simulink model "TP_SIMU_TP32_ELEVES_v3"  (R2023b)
settings: Solver=ode15s  StartTime=0.0  StopTime=6  RelTol=1e-3  EnableMultiTasking=on
libraries: fl_lib x24, nesl_utility x12, sdl_lib x2

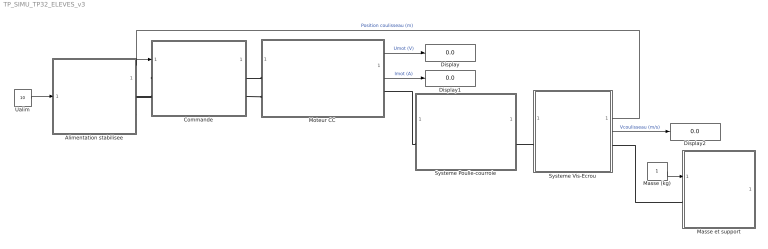
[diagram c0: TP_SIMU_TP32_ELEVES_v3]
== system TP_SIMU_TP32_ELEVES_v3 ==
  Alimentation stabilisee : Subsystem
  Commande : Subsystem
  Display : Display
  Display1 : Display
  Display2 : Display
  Masse (kg) : Constant
  Masse et support : Subsystem
  Moteur CC : Subsystem
  Systeme Poulie-courroie : Subsystem  mask{rend=0.64}
      mask prompts: rend "Rendement"
  Systeme Vis-Ecrou : Subsystem
  Ualim : Constant  Value=10
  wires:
  Masse (kg)/1 -> Masse et support/1(In1)
  Systeme Vis-Ecrou/1(Position coulisseau) -> Commande/1(In1)  "Position coulisseau (m)"
  Ualim/1 -> Alimentation stabilisee/1(Ualim)
  Moteur CC/1(Umot) -> Display/1  "Umot (V)"
  Moteur CC/2(Imot) -> Display1/1  "Imot (A)"
  Systeme Vis-Ecrou/2(Vcoulisseau) -> Display2/1  "Vcoulisseau (m/s)"
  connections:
  Systeme Poulie-courroie/LConn1 -- Moteur CC/RConn1
  Commande/RConn1 -- Moteur CC/LConn1
  Commande/LConn1 -- Alimentation stabilisee/RConn1
  Alimentation stabilisee/RConn2 -- Commande/LConn2
  Commande/RConn2 -- Moteur CC/LConn2
  Systeme Vis-Ecrou/LConn1 -- Systeme Poulie-courroie/RConn1
  Masse et support/LConn1 -- Systeme Vis-Ecrou/RConn1

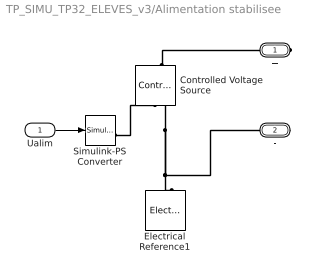
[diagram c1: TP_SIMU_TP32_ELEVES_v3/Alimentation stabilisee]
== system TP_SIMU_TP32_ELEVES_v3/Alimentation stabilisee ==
  Ualim : Inport
  Controlled Voltage Source : fl_lib/Electrical/Electrical Sources/Controlled Voltage Source
  Electrical Reference1 : fl_lib/Electrical/Electrical Elements/Electrical Reference
  Simulink-PS Converter : nesl_utility/Simulink-PS Converter  PhysicalDomain=network_engine_domain  SubClassName=ps_input  LeftPortType=input  RightPortType=output  PseudoPeriodic=off  Frequencies=[]  NoiseDistribution=none  NoiseParameters=[]  Unit=1  AffineConversion=off  FilteringAndDerivatives=provide  SimscapeFilterOrder=1  InputFilterTimeConstant=0.001  UdotUserProvided=0
  + : PMIOPort  Side=Right
  - : PMIOPort  Port=2  Side=Right
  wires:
  Ualim/1 -> Simulink-PS Converter/1
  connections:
  Controlled Voltage Source/LConn1 -- +/RConn1
  Electrical Reference1/LConn1 -- Controlled Voltage Source/RConn2 -- -/RConn1
  Simulink-PS Converter/RConn1 -- Controlled Voltage Source/RConn1

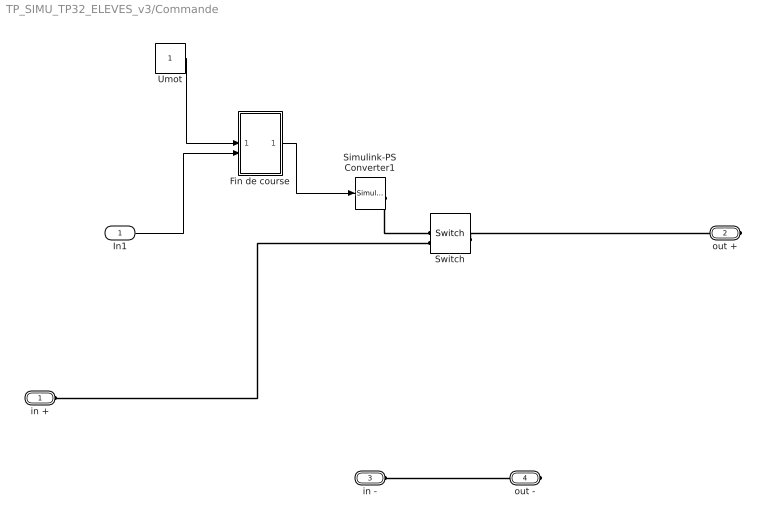
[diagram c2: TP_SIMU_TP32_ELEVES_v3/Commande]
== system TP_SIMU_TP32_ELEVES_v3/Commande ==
  In1 : Inport
  Fin de course : Subsystem
  Simulink-PS Converter1 : nesl_utility/Simulink-PS Converter  PhysicalDomain=network_engine_domain  SubClassName=ps_input  LeftPortType=input  RightPortType=output  PseudoPeriodic=off  Frequencies=[]  NoiseDistribution=none  NoiseParameters=[]  Unit=V  AffineConversion=off  FilteringAndDerivatives=zero  SimscapeFilterOrder=1  InputFilterTimeConstant=.001  UdotUserProvided=0
  Switch : fl_lib/Electrical/Electrical Elements/Switch  R_closed=0.01 Ohm  G_open=1e-8 1/Ohm  Threshold=0  i_specify=off  i_priority=None  i=0 A  i_nominal_specify=off  i_nominal_unit=A  i_nominal_value=1  v_specify=off  v_priority=None  v=0 V  v_nominal_specify=off  v_nominal_unit=V  v_nominal_value=1
  Umot : Constant
  in + : PMIOPort  Side=Left
  out + : PMIOPort  Port=2  Side=Right
  in - : PMIOPort  Port=3  Side=Left
  out - : PMIOPort  Port=4  Side=Right
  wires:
  Umot/1 -> Fin de course/1(In1)
  In1/1 -> Fin de course/2(In2)
  Fin de course/1(Out1) -> Simulink-PS Converter1/1
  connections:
  Switch/RConn2 -- in +/RConn1
  Simulink-PS Converter1/RConn1 -- Switch/RConn1
  Switch/LConn1 -- out +/RConn1
  in -/RConn1 -- out -/RConn1

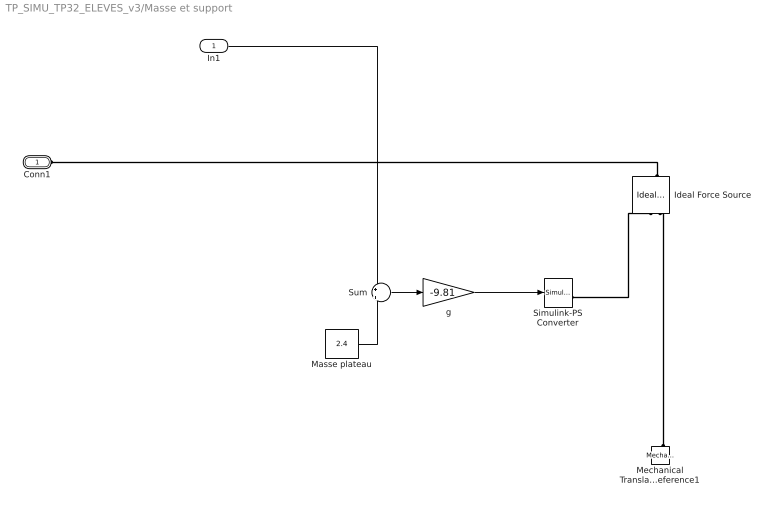
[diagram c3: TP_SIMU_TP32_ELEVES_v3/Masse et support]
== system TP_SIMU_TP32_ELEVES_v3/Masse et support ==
  In1 : Inport
  Ideal Force Source : fl_lib/Mechanical/Mechanical Sources/Ideal Force Source
  Masse plateau : Constant  Value=2.4
  Mechanical Translational Reference1 : fl_lib/Mechanical/Translational Elements/Mechanical Translational Reference
  Simulink-PS Converter : nesl_utility/Simulink-PS Converter  PhysicalDomain=network_engine_domain  SubClassName=ps_input  LeftPortType=input  RightPortType=output  PseudoPeriodic=off  Frequencies=[]  NoiseDistribution=none  NoiseParameters=[]  Unit=1  AffineConversion=off  FilteringAndDerivatives=zero  SimscapeFilterOrder=1  InputFilterTimeConstant=.001  UdotUserProvided=0
  Sum : Sum  Inputs=+|+
  g : Gain  Gain=-9.81
  Conn1 : PMIOPort  Side=Left
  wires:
  g/1 -> Simulink-PS Converter/1
  Sum/1 -> g/1
  Masse plateau/1 -> Sum/2
  In1/1 -> Sum/1
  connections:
  Mechanical Translational Reference1/LConn1 -- Ideal Force Source/RConn2
  Ideal Force Source/LConn1 -- Conn1/RConn1
  Simulink-PS Converter/RConn1 -- Ideal Force Source/RConn1

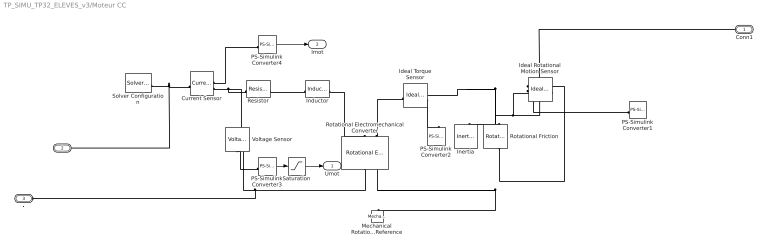
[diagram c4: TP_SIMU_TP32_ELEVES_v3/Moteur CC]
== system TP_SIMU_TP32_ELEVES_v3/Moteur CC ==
  Current Sensor : fl_lib/Electrical/Electrical Sensors/Current Sensor
  Ideal Rotational Motion Sensor : fl_lib/Mechanical/Mechanical Sensors/Ideal Rotational Motion Sensor  reference=foundation.enum.MeasurementReference.difference  acceleration_port=false  velocity_port=true  position_port=true  wrap_angle=false  offset=0 rad
  Ideal Torque Sensor : fl_lib/Mechanical/Mechanical Sensors/Ideal Torque Sensor
  Inductor : fl_lib/Electrical/Electrical Elements/Inductor  l=2e-4 H  r=0 Ohm  g=1e-9 1/Ohm  i_specify=off  i_priority=None  i=0 A  i_nominal_specify=off  i_nominal_unit=A  i_nominal_value=1  v_specify=off  v_priority=None  v=0 V  v_nominal_specify=off  v_nominal_unit=V  v_nominal_value=1  i_L_specify=on  i_L_priority=High  i_L=0 A  i_L_nominal_specify=off  i_L_nominal_unit=A  i_L_nominal_value=1
  Inertia : fl_lib/Mechanical/Rotational Elements/Inertia  inertia=5e-5 kg*m^2  num_ports=foundation.enum.numPorts2.one  w_specify=on  w_priority=High  w=0 rad/s  w_nominal_specify=off  w_nominal_unit=rad/s  w_nominal_value=1  t_specify=off  t_priority=None  t=0 N*m  t_nominal_specify=off  t_nominal_unit=N*m  t_nominal_value=1
  Mechanical Rotational Reference : fl_lib/Mechanical/Rotational Elements/Mechanical Rotational Reference
  PS-Simulink Converter1 : nesl_utility/PS-Simulink Converter  PhysicalDomain=network_engine_domain  SubClassName=ps_output  LeftPortType=input  RightPortType=output  PseudoPeriodic=off  Frequencies=[]  VectorFormat=1-D array  Unit=rad/s  AffineConversion=off
  PS-Simulink Converter2 : nesl_utility/PS-Simulink Converter  PhysicalDomain=network_engine_domain  SubClassName=ps_output  LeftPortType=input  RightPortType=output  PseudoPeriodic=off  Frequencies=[]  VectorFormat=1-D array  Unit=N*m  AffineConversion=off
  PS-Simulink Converter3 : nesl_utility/PS-Simulink Converter  PhysicalDomain=network_engine_domain  SubClassName=ps_output  LeftPortType=input  RightPortType=output  PseudoPeriodic=off  Frequencies=[]  VectorFormat=1-D array  Unit=V  AffineConversion=off
  PS-Simulink Converter4 : nesl_utility/PS-Simulink Converter  PhysicalDomain=network_engine_domain  SubClassName=ps_output  LeftPortType=input  RightPortType=output  PseudoPeriodic=off  Frequencies=[]  VectorFormat=1-D array  Unit=A  AffineConversion=off
  Resistor : fl_lib/Electrical/Electrical Elements/Resistor  R=1.8 Ohm  i_specify=off  i_priority=None  i=0 A  i_nominal_specify=off  i_nominal_unit=A  i_nominal_value=1  v_specify=off  v_priority=None  v=0 V  v_nominal_specify=off  v_nominal_unit=V  v_nominal_value=1
  Rotational Electromechanical Converter : fl_lib/Electrical/Electrical Elements/Rotational Electromechanical Converter  K=0.019 V/(rad/s)  i_specify=off  i_priority=None  i=0 A  i_nominal_specify=off  i_nominal_unit=A  i_nominal_value=1  v_specify=off  v_priority=None  v=0 V  v_nominal_specify=off  v_nominal_unit=V  v_nominal_value=1  t_specify=off  t_priority=None  t=0 N*m  t_nominal_specify=off  t_nominal_unit=N*m  t_nominal_value=1  w_specify=off  w_priority=None  w=0 rad/s  w_nominal_specify=off  w_nominal_unit=rad/s  w_nominal_value=1
  Rotational Friction : fl_lib/Mechanical/Rotational Elements/Rotational Friction  brkwy_trq=1.2e-2 N*m  brkwy_vel=0.060623 rad/s  Col_trq=1.2e-2 N*m  visc_coef=5e-9 N*m/(rad/s)  w_specify=off  w_priority=None  w=0 rad/s  w_nominal_specify=off  w_nominal_unit=rad/s  w_nominal_value=1  t_specify=off  t_priority=None  t=0 N*m  t_nominal_specify=off  t_nominal_unit=N*m  t_nominal_value=1
  Saturation : Saturate  UpperLimit=20
  Solver Configuration : nesl_utility/Solver Configuration  PhysicalDomain=network_engine_domain  SubClassName=solver  LeftPortType=input  RightPortType=generic  Tones=[]  Harmonics=[]  SimulateNoise=off  Profile=off  UseLocalSampling=off  EnableSwitchedLinearOptims=on  FrequencyDomain=off  UseCCode=off  RelTol=0.001  AbsTol=1e-06  MinStep=1e-09  ToWorkspace=off  RevertToSquareIcSolve=off  NumHomotopyIterations=100  PhasorMode=off  PhasorModeNumHarmonics=1  ConsistencySolver=NEWTON_FTOL  IndexReductionMethod=DerivativeReplacement  DoDC=off  ResidualTolerance=1e-9  ConsistencyTolSource=GLOBAL  ConsistencyAbsTol=0.001  ConsistencyRelTol=0.001  ConsistencyTolFactor=0.001  UseLocalSolver=off  LocalSolverChoice=NE_BACKWARD_EULER_ADVANCER  ResolveIndetEquations=on  FunctionEvalNumThread=1  LocalSolverSampleTime=.001  DoFixedCost=off  MaxNonlinIter=3  MaxModeIter=2  ComputeImpulses=off  ImpulseIterations=2  LinearAlgebra=Sparse  LinearAlgebraNumThread=0  EquationFormulation=NE_TIME_EF  DelaysMemoryBudget=1024  AutomaticFiltering=on  FilteringTimeConstant=0.001  PartitionStorageMethod=AS_NEEDED  PartitionMemoryBudget=1024  PartitionMethod=FAST  MultibodyUseLocalSolver=off  MultibodyLocalSolverChoice=ODE1  MultibodyLocalSolverSampleTime=0.001
  Voltage Sensor : fl_lib/Electrical/Electrical Sensors/Voltage Sensor
  Conn1 : PMIOPort  Side=Right
  + : PMIOPort  Port=2  Side=Left
  - : PMIOPort  Port=3  Side=Left
  Umot : Outport  VectorParamsAs1DForOutWhenUnconnected=off
  Imot : Outport  Port=2  VectorParamsAs1DForOutWhenUnconnected=off
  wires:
  PS-Simulink Converter3/1 -> Saturation/1
  PS-Simulink Converter4/1 -> Imot/1
  Saturation/1 -> Umot/1
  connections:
  Ideal Rotational Motion Sensor/RConn2 -- PS-Simulink Converter1/LConn1
  Current Sensor/RConn1 -- PS-Simulink Converter4/LConn1
  Rotational Friction/RConn1 -- Rotational Electromechanical Converter/RConn2 -- Mechanical Rotational Reference/LConn1 -- Ideal Rotational Motion Sensor/RConn1
  Inductor/RConn1 -- Rotational Electromechanical Converter/LConn1
  Ideal Torque Sensor/RConn2 -- PS-Simulink Converter2/LConn1
  Rotational Electromechanical Converter/LConn2 -- Ideal Torque Sensor/LConn1
  Solver Configuration/RConn1 -- +/RConn1 -- Current Sensor/LConn1
  Resistor/RConn1 -- Inductor/LConn1
  Rotational Friction/LConn1 -- Ideal Torque Sensor/RConn1 -- Inertia/LConn1 -- Conn1/RConn1 -- Ideal Rotational Motion Sensor/LConn1
  Current Sensor/RConn2 -- Voltage Sensor/LConn1 -- Resistor/LConn1
  Rotational Electromechanical Converter/RConn1 -- Voltage Sensor/RConn2 -- -/RConn1
  PS-Simulink Converter3/LConn1 -- Voltage Sensor/RConn1

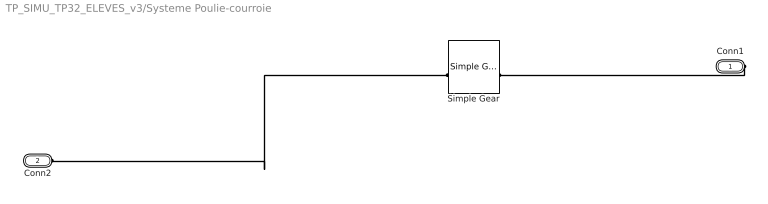
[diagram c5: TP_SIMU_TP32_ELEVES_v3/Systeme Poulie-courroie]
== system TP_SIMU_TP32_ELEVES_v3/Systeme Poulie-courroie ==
  Simple Gear : sdl_lib/Gears/Simple Gear  ratio=71/20  rotation_direction=3-2*(1)  friction_model=sdl.enum.gear_efficiencies_load.constant  T_noload=0.1 N*m  T_nom=5 N*m  efficiency_nom=0.8  efficiency=rend  temperature_TLU=[280, 300, 320] K  load_TLU=[1, 5, 10] N*m  efficiency_TLU=[.95, .9, .85]  efficiency_TLU2=[.85, .8, .75; .95, .9, .85; .85, .8, .7]  w_thr=0.01 rad/s  pwr_thr=0.001 W  enable_backlash=false  hardstop_model=simscape.enum.hardstop.smooth  backlash_distance=1e-3 mm  r_base=0.1 m  transition=1e-4 mm  backlash_stiffness=1e6 N/m  backlash_damping=1e3 N*s/m  coeff_rest=0.7  v_tol=0.001 m/s  f_tol=0 N  mu_visc=[ 0 0 ] N*m/(rad/s)  enable_faults=simscape.enum.onoff.off  efficiency_fault=0.05  external_fault=simscape.enum.onoff.off  temporal_fault=simscape.enum.onoff.off  fault_time=5 s  fault_angles=pi / 12 rad  report_fault=(1)-1  thermal_mass=50 J/K  temperature_specify=off  temperature_priority=High  temperature=300 K  temperature_nominal_specify=off  temperature_nominal_unit=K  temperature_nominal_value=1  x_backlash_specify=off  x_backlash_priority=None  x_backlash=0 mm  x_backlash_nominal_specify=off  x_backlash_nominal_unit=mm  x_backlash_nominal_value=1  f_hardstop_specify=off  f_hardstop_priority=None  f_hardstop=0 N  f_hardstop_nominal_specify=off  f_hardstop_nominal_unit=N  f_hardstop_nominal_value=1  v_backlash_specify=off  v_backlash_priority=None  v_backlash=0 m/s  v_backlash_nominal_specify=off  v_backlash_nominal_unit=m/s  v_backlash_nominal_value=1
  Conn1 : PMIOPort  Side=Right
  Conn2 : PMIOPort  Port=2  Side=Left
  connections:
  Conn1/RConn1 -- Simple Gear/RConn1
  Simple Gear/LConn1 -- Conn2/RConn1

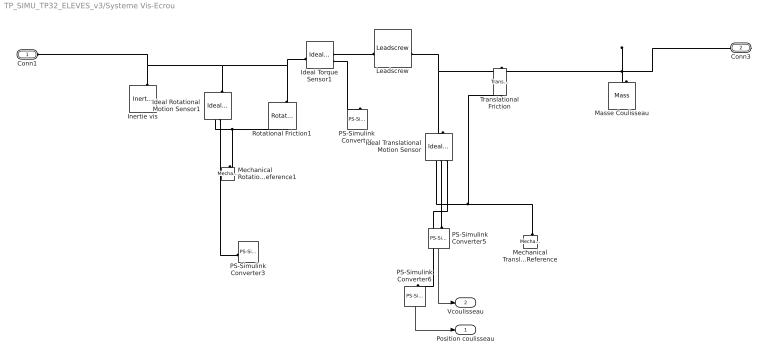
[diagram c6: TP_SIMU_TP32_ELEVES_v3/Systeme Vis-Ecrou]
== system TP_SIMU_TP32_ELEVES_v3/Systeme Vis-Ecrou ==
  Ideal Rotational Motion Sensor1 : fl_lib/Mechanical/Mechanical Sensors/Ideal Rotational Motion Sensor  reference=foundation.enum.MeasurementReference.difference  acceleration_port=false  velocity_port=true  position_port=true  wrap_angle=false  offset=0 rad
  Ideal Torque Sensor1 : fl_lib/Mechanical/Mechanical Sensors/Ideal Torque Sensor
  Ideal Translational Motion Sensor : fl_lib/Mechanical/Mechanical Sensors/Ideal Translational Motion Sensor  reference=foundation.enum.MeasurementReference.difference  acceleration_port=false  velocity_port=true  position_port=true  offset=0 m
  Inertie vis : fl_lib/Mechanical/Rotational Elements/Inertia  inertia=1e-5 kg*m^2  num_ports=foundation.enum.numPorts2.one  w_specify=on  w_priority=High  w=0 rad/s  w_nominal_specify=off  w_nominal_unit=rad/s  w_nominal_value=1  t_specify=off  t_priority=None  t=0 N*m  t_nominal_specify=off  t_nominal_unit=N*m  t_nominal_value=1
  Leadscrew : sdl_lib/Gears/Rotational- Translational/Leadscrew  Lead=3 mm  helix_type=1  friction_model=2  friction_parameterization=2  lambda=15 deg  alpha=14.5 deg  fr_coeff=0.08  eff_sn=0.5  eff_ns=0  temperature_TLU=[280, 300, 320] K  efficiency_sn_TLU=[.75, .65, .6]  efficiency_ns_TLU=[.5, .45, .4]  pwr_thr=0.001 W  mu_visc=0 N*m/(rad/s)  thermal_mass=50 J/K  temperature_specify=off  temperature_priority=High  temperature=300 K  temperature_nominal_specify=off  temperature_nominal_unit=K  temperature_nominal_value=1
  Masse Coulisseau : fl_lib/Mechanical/Translational Elements/Mass  mass=0.145203 kg  num_ports=foundation.enum.numPorts2.one  v_specify=on  v_priority=High  v=0 m/s  v_nominal_specify=off  v_nominal_unit=m/s  v_nominal_value=1  f_specify=off  f_priority=None  f=0 N  f_nominal_specify=off  f_nominal_unit=N  f_nominal_value=1
  Mechanical Rotational Reference1 : fl_lib/Mechanical/Rotational Elements/Mechanical Rotational Reference
  Mechanical Translational Reference : fl_lib/Mechanical/Translational Elements/Mechanical Translational Reference
  PS-Simulink Converter{,3,5..6} (4 alike) : nesl_utility/PS-Simulink Converter  PhysicalDomain=network_engine_domain  SubClassName=ps_output  LeftPortType=input  RightPortType=output  PseudoPeriodic=off  Frequencies=[]  VectorFormat=1-D array  Unit=1  AffineConversion=off
  Rotational Friction1 : fl_lib/Mechanical/Rotational Elements/Rotational Friction  brkwy_trq=0.01 N*m  brkwy_vel=0.060623 rad/s  Col_trq=0.01 N*m  visc_coef=0 N*m/(rad/s)  w_specify=off  w_priority=None  w=0 rad/s  w_nominal_specify=off  w_nominal_unit=rad/s  w_nominal_value=1  t_specify=off  t_priority=None  t=0 N*m  t_nominal_specify=off  t_nominal_unit=N*m  t_nominal_value=1
  Translational Friction : fl_lib/Mechanical/Translational Elements/Translational Friction  brkwy_frc=1 N  brkwy_vel=0.060623 m/s  Col_frc=1 N  visc_coef=0 N/(m/s)  v_specify=off  v_priority=None  v=0 m/s  v_nominal_specify=off  v_nominal_unit=m/s  v_nominal_value=1  f_specify=off  f_priority=None  f=0 N  f_nominal_specify=off  f_nominal_unit=N  f_nominal_value=1
  Conn1 : PMIOPort  Side=Left
  Conn3 : PMIOPort  Port=2  Side=Right
  Position coulisseau : Outport  VectorParamsAs1DForOutWhenUnconnected=off
  Vcoulisseau : Outport  Port=2  VectorParamsAs1DForOutWhenUnconnected=off
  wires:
  PS-Simulink Converter5/1 -> Vcoulisseau/1
  PS-Simulink Converter6/1 -> Position coulisseau/1
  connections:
  Ideal Translational Motion Sensor/RConn2 -- PS-Simulink Converter5/LConn1
  Ideal Rotational Motion Sensor1/RConn2 -- PS-Simulink Converter3/LConn1
  Ideal Torque Sensor1/RConn1 -- Leadscrew/LConn1
  Ideal Torque Sensor1/RConn2 -- PS-Simulink Converter/LConn1
  Ideal Translational Motion Sensor/RConn3 -- PS-Simulink Converter6/LConn1
  Masse Coulisseau/LConn1 -- Conn3/RConn1 -- Leadscrew/RConn1 -- Ideal Translational Motion Sensor/LConn1 -- Translational Friction/LConn1
  Translational Friction/RConn1 -- Ideal Translational Motion Sensor/RConn1 -- Mechanical Translational Reference/LConn1
  Inertie vis/LConn1 -- Conn1/RConn1 -- Ideal Torque Sensor1/LConn1 -- Rotational Friction1/LConn1 -- Ideal Rotational Motion Sensor1/LConn1
  Rotational Friction1/RConn1 -- Ideal Rotational Motion Sensor1/RConn1 -- Mechanical Rotational Reference1/LConn1

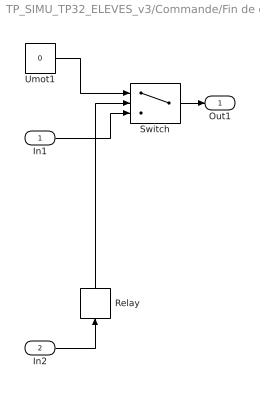
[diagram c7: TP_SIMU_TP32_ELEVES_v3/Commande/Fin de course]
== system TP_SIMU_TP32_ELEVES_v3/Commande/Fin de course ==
  In1 : Inport
  In2 : Inport  Port=2
  Relay : Relay  OnSwitchValue=0.25  OffSwitchValue=0
  Switch : Switch  Threshold=1
  Umot1 : Constant  Value=0
  Out1 : Outport  VectorParamsAs1DForOutWhenUnconnected=off
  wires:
  Umot1/1 -> Switch/1
  Relay/1 -> Switch/2
  Switch/1 -> Out1/1
  In1/1 -> Switch/3
  In2/1 -> Relay/1
